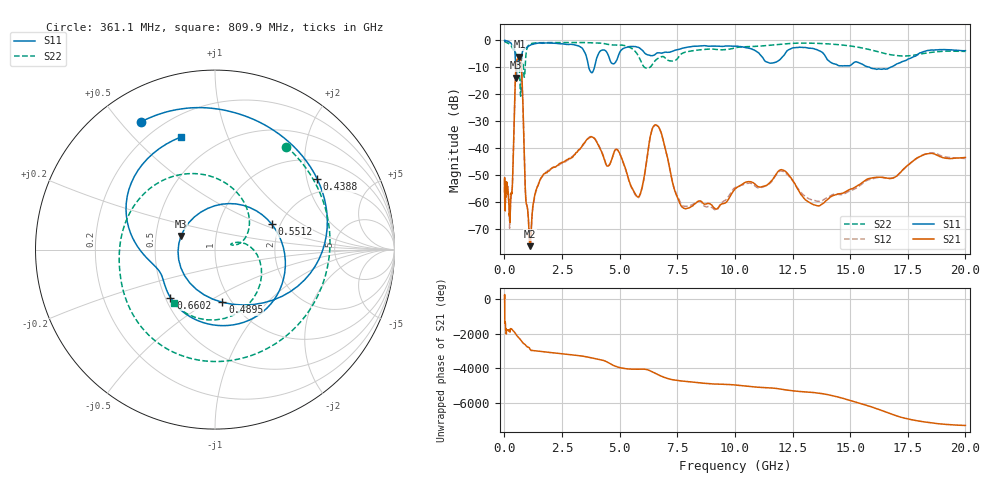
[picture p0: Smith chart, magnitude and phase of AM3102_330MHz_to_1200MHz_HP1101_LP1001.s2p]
! Date/Time: Tue, Sep 11, 2018 5:22 PM
! Network Analyzer: Agilent Technologies E8362B Rev: A.07.50.63
! Sweep from 0.010 to 20.000 GHz, 1601 Points, Sweep Type: LOG
! Power Supply: 4.949 V, 0.001 A
# Hz S DB R 50
!freq MagS11 AngS11 MagS21 AngS21 MagS12 AngS12 MagS22 AngS22
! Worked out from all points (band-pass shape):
!   1601 points, 10 MHz to 20 GHz, reference 50 ohm
!   highest |S21| = -5.99 dB at 650.9 MHz (marker M1); lowest = -76.2 dB at 1.119 GHz (marker M2)
!   |S21| within 3 dB of the highest: 508 MHz to 730.1 MHz (222.1 MHz wide, 35.9 % of centre)
!   lowest |S11| = -13.8 dB at 513.3 MHz (marker M3), VSWR 1.51, Z = 33.7 + j5.36 ohm
!   |S11| at or under -10 dB: 487.5 MHz to 543.6 MHz (56.07 MHz wide, 10.9 % of centre); 3.663 GHz to 3.906 GHz (243.4 MHz wide, 6.43 % of centre); 15.86 GHz to 16.74 GHz (879.8 MHz wide, 5.4 % of centre)
!   |S22| runs from -20.6 to -0.2 dB; largest |S21 - S12| = 0.0089
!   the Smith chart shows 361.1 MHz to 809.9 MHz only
!   S11 on the Smith chart (normalised r, x): 361.1 MHz: 0.13, +0.57; 438.8 MHz: 1.54, +2.32; 489.5 MHz: 0.91, -0.58; 551.2 MHz: 1.80, +0.58; 660.2 MHz: 0.53, -0.33; 809.9 MHz: 0.32, +0.69
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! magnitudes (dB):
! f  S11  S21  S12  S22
! 10 MHz  0.0  -56.2  -51.6  -0.3
! 35.55 MHz  -0.1  -56.9  -57.4  -0.4
! 126.4 MHz  -0.2  -55.1  -53.8  -0.9
! 227.8 MHz  -0.7  -64.8  -69.5  -1.3
! 361.1 MHz  -1.7  -50.7  -51.3  -3.1
! 438.8 MHz  -3.2  -24.9  -25.0  -4.1
! 447.2 MHz  -3.6  -22.4  -22.4  -4.1
! 489.5 MHz  -10.6  -11.6  -11.6  -4.7
! 513.3 MHz  -13.8  -8.5  -8.6  -5.3
! 551.2 MHz  -9.2  -7.2  -7.1  -5.7
! 650.9 MHz  -8.4  -6.0  -6.0  -11.0
! 660.2 MHz  -8.8  -6.0  -6.0  -12.4
! 809.9 MHz  -3.7  -25.2  -25.3  -8.5
! 920.7 MHz  -2.9  -57.5  -57.5  -6.8
! 1.119 GHz  -1.8  -76.2  -75.1  -1.3
! 1.59 GHz  -1.0  -50.9  -50.9  -0.8
! 3.775 GHz  -11.9  -35.7  -35.6  -0.8
! 5.652 GHz  -2.2  -56.5  -56.8  -3.8
! 6.58 GHz  -4.9  -31.3  -31.4  -7.2
! 7.92 GHz  -2.5  -62.2  -61.4  -4.2
! 13.61 GHz  -3.7  -61.3  -59.5  -1.1
! 20 GHz  -3.8  -43.3  -43.7  -4.0
